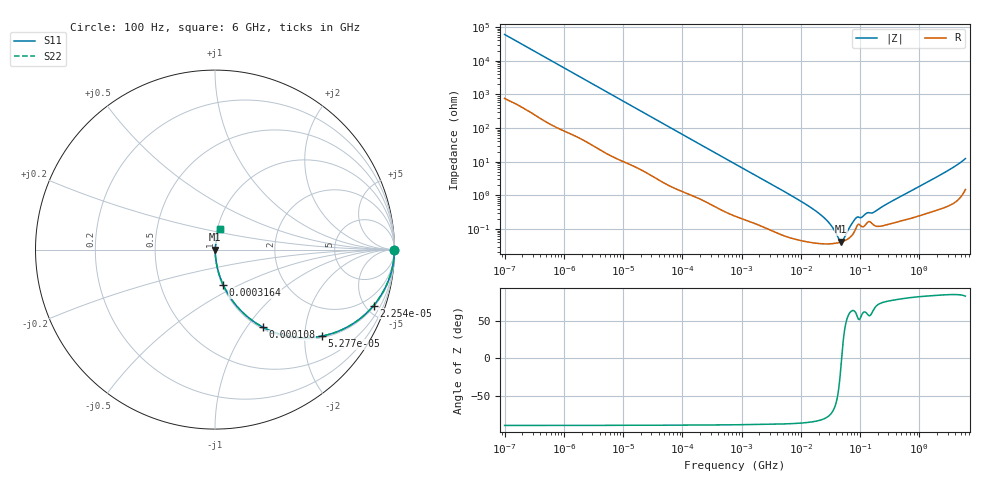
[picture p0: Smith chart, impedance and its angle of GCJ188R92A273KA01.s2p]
!Murata Part Number: GCJ188R92A273KA01
!These Parameters are Measured in Series Mode Connection
!Data Generated on Mar 13, 2026
!  o--ll--o
!Port1  Port2
!  o------o
!Operation Temp=25[degC], DC Bias Voltage=0[V]
!Freq. Start=100[Hz] Stop=6[GHz] 401[Steps]
# Hz S RI R 50
!Freq.(Hz) S11(Real) S11(Imag) S21(Real) S21(Imag) S12(Real) S12(Imag) S22(Real) S22(Imag)
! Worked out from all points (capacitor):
!   401 points, 100 Hz to 6 GHz, reference 50 ohm
!   read as one part in series: C = 26.3 nF near 109 Hz
!   lowest |Z| = 41.5 mohm at 47.65 MHz (marker M1)
!   series resonance near 48.84 MHz, so ESL is about 400 pH
!   S11 on the Smith chart (normalised r, x): 100 Hz: open; 22.54 kHz: 1.10, -5.63; 52.77 kHz: 1.04, -2.43; 108 kHz: 1.02, -1.19; 316.4 kHz: 1.01, -0.41; 6 GHz: 1.03, +0.25
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100  1 -0.00166  2.36e-05 0.00166  2.36e-05 0.00166  1 -0.00166
2008  0.9985 -0.0324  0.00153 0.0324  0.00153 0.0324  0.9985 -0.0324
7695  0.9834 -0.1205  0.0166 0.1205  0.0166 0.1205  0.9834 -0.1205
22537  0.8836 -0.3118  0.1164 0.3118  0.1164 0.3118  0.8836 -0.3118
40335  0.7116 -0.4442  0.2884 0.4442  0.2884 0.4442  0.7116 -0.4442
52766  0.5941 -0.4822  0.4059 0.4822  0.4059 0.4822  0.5941 -0.4822
108014  0.2671 -0.4323  0.7329 0.4323  0.7329 0.4323  0.2671 -0.4323
176758  0.1247 -0.3189  0.8753 0.3189  0.8753 0.3189  0.1247 -0.3189
316350  0.0457 -0.1968  0.9543 0.1968  0.9543 0.1968  0.0457 -0.1968
774597  0.00963 -0.0846  0.9904 0.0846  0.9904 0.0846  0.00963 -0.0846
1.555665e7  0.000407 -0.00405  0.9996 0.00405  0.9996 0.00405  0.000407 -0.00405
2.911731e7  0.000362 -0.00157  0.9996 0.00157  0.9996 0.00157  0.000362 -0.00157
4.35672e7  0.000392 -0.000337  0.9996 0.000337  0.9996 0.000337  0.000392 -0.000337
4.764863e7  0.000408 -7.27e-05  0.9996 7.27e-05  0.9996 7.27e-05  0.000408 -7.27e-05
5.211241e7  0.000431 0.000195  0.9996 -0.000195  0.9996 -0.000195  0.000431 0.000195
6.817316e7  0.000569 0.00105  0.9994 -0.00105  0.9994 -0.00105  0.000569 0.00105
8.527865e7  0.00105 0.00183  0.999 -0.00183  0.999 -0.00183  0.00105 0.00183
1.334425e8  0.00157 0.00259  0.9984 -0.00259  0.9984 -0.00259  0.00157 0.00259
1.745687e8  0.00128 0.00294  0.9987 -0.00294  0.9987 -0.00294  0.00128 0.00294
3.124326e8  0.00143 0.00593  0.9986 -0.00593  0.9986 -0.00593  0.00143 0.00593
2.450438e9  0.00594 0.043  0.9941 -0.043  0.9941 -0.043  0.00594 0.043
6e9  0.0289 0.1174  0.9711 -0.1174  0.9711 -0.1174  0.0289 0.1174
